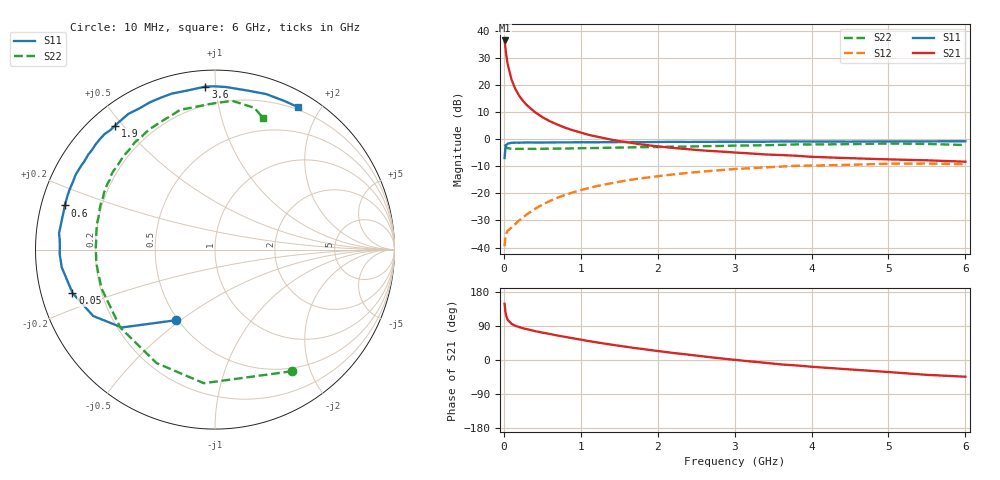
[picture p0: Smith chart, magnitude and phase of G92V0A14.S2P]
! SIEMENS Small Signal Semiconductors
! BFG235
! Si NPN RF Bipolar Junction Transistor in SOT223
! VCE = 2 V  IC = 140 mA
! Common Emitter S-Parameters:  July  1994
# GHz  S  MA  R  50
!  f  S11  S21  S12  S22
! GHz  MAG  ANG  MAG  ANG  MAG  ANG  MAG  ANG
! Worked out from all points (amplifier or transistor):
!   40 points, 10 MHz to 6 GHz, reference 50 ohm
!   highest |S21| = 36.5 dB at 10 MHz (marker M1)
!   |S21| within 3 dB of that: start of sweep to 21.67 MHz
!   unconditionally stable (mu >= 1): 428.7 MHz to 1.611 GHz; 1.753 GHz to 1.914 GHz
!   at 200 MHz: K = 0.82, MSG = 23.0 dB, |S12| = -30.0 dB
!   at 1.5 GHz: K = 1.01, MAG = 6.9 dB, |S12| = -15.7 dB
!   at 6 GHz: K = 0.93, MSG = 0.5 dB, |S12| = -9.2 dB
!   S11 on the Smith chart (normalised r, x): 10 MHz: 0.49, -0.48; 50 MHz: 0.09, -0.15; 600 MHz: 0.07, +0.14; 1.9 GHz: 0.07, +0.48; 3.6 GHz: 0.09, +0.94; 6 GHz: 0.17, +1.72
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0.01  0.45 -119.0  66.78 148.1  0.0106 57.6  0.8025 -57.6
0.02  0.6764 -140.1  49.54 128.3  0.0159 43.2  0.747 -94.8
0.03  0.773 -151.4  37.49 117.1  0.0181 36.8  0.711 -117.3
0.05  0.8299 -163.1  24.3 105.9  0.0204 31.2  0.6836 -140.5
0.1  0.8597 -173.4  12.65 95.5  0.0234 35.9  0.6683 -161.1
0.15  0.8657 -178.4  8.463 90.2  0.0273 43.4  0.6637 -169.4
0.2  0.8646 178.9  6.327 86.8  0.0318 48.4  0.6654 -174.0
0.25  0.8671 176.3  5.095 83.7  0.0362 51.9  0.6633 -177.3
0.3  0.8737 174.0  4.254 81.3  0.041 55.3  0.6646 179.9
0.4  0.8696 169.9  3.203 76.5  0.0514 58.3  0.6639 176.0
0.5  0.8692 166.4  2.564 72.3  0.0619 59.6  0.6669 172.8
0.6  0.8724 163.6  2.146 68.7  0.0727 59.7  0.6702 169.7
0.8  0.8766 157.2  1.628 60.9  0.0942 58.3  0.6737 164.3
1.1  0.8799 148.1  1.21 50.0  0.1251 54.2  0.687 157.2
1.5  0.8867 138.6  0.922 37.5  0.164 47.2  0.7027 148.3
1.9  0.8871 128.9  0.766 26.3  0.1991 39.8  0.7168 140.1
2.2  0.8971 122.5  0.692 18.6  0.2237 34.0  0.7294 134.3
3.2  0.8993 101.5  0.547 -3.7  0.2921 14.6  0.7678 115.5
3.6  0.9099 93.4  0.511 -11.6  0.3128 6.3  0.7879 107.4
4.5  0.9045 78.3  0.447 -24.9  0.3377 -9.4  0.8121 91.9
5.5  0.9134 65.5  0.408 -39.2  0.3563 -26.9  0.8196 74.5
6  0.919 59.9  0.385 -44.1  0.346 -33.5  0.7816 70.0
